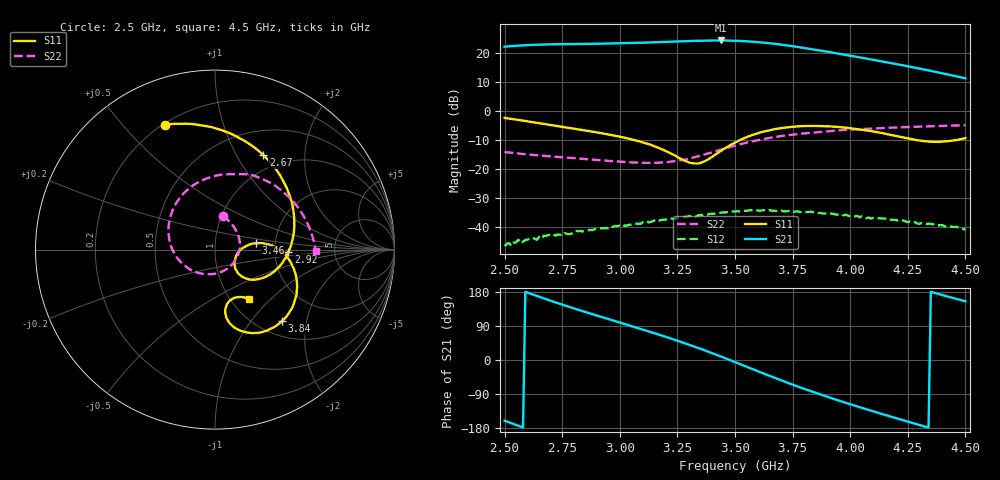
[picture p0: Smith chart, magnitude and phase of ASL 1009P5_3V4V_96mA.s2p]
!ASL 1009P5 : Low Noise Amplifier S-parameter data 2.5-4.5 GHz
!Bias conditions Vd1=3V, Vd2=4V, Total current=96 mA
!Date: Tuesday, January 09, 2007 14:22:50
!S2P File: Measurements: S11, S21, S12, S22:
# Hz S  dB  R 50
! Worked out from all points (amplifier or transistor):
!   201 points, 2.5 GHz to 4.5 GHz, reference 50 ohm
!   highest |S21| = 24.2 dB at 3.44 GHz (marker M1)
!   |S21| within 3 dB of that: start of sweep to 3.833 GHz
!   unconditionally stable (mu >= 1): start of sweep to end of sweep
!   at 2.83 GHz: K = 3.30, MAG = 24.1 dB, |S12| = -41.4 dB
!   at 3.5 GHz: K = 1.64, MAG = 24.8 dB, |S12| = -34.8 dB
!   at 4.5 GHz: K = 9.42, MAG = 13.4 dB, |S12| = -41.1 dB
!   S11 on the Smith chart (normalised r, x): 2.5 GHz: 0.21, +0.66; 2.67 GHz: 0.80, +1.30; 2.92 GHz: 2.38, -0.08; 3.46 GHz: 1.58, +0.12; 3.84 GHz: 1.27, -1.44; 4.5 GHz: 1.21, -0.76
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2.5e9  -2.51 111.8  22.06 -160.3  -46.71 121.9  -14.25 76.8
2.59e9  -3.56 86.0  22.57 179.8  -44.59 102.7  -15.02 64.5
2.67e9  -4.56 62.9  22.81 162.7  -43.10 85.0  -15.55 53.0
2.74e9  -5.46 43.3  22.93 148.3  -42.76 70.6  -16.01 42.3
2.84e9  -6.70 17.0  23.01 128.7  -41.67 56.2  -16.60 24.0
2.92e9  -7.76 -1.9  23.09 113.7  -40.51 42.8  -17.14 7.8
3.04e9  -9.65 -26.1  23.31 91.5  -39.32 22.0  -17.77 -22.7
3.17e9  -12.88 -43.9  23.64 66.9  -37.97 -1.4  -17.97 -64.6
3.25e9  -15.97 -43.7  23.88 50.9  -36.86 -15.6  -17.28 -95.1
3.31e9  -18.04 -28.5  24.04 38.3  -36.29 -29.0  -16.34 -118.3
3.38e9  -16.93 -0.6  24.17 22.9  -35.83 -41.8  -14.82 -144.9
3.44e9  -13.81 8.8  24.21 9.0  -35.13 -57.1  -13.39 -166.6
3.46e9  -12.79 8.9  24.18 4.2  -35.08 -60.9  -12.92 -173.5
3.5e9  -10.97 6.6  24.12 -5.5  -34.78 -69.8  -12.03 173.1
3.58e9  -8.26 -3.7  23.76 -25.0  -34.60 -90.2  -10.49 148.2
3.67e9  -6.40 -18.8  23.08 -46.7  -34.50 -111.7  -9.09 123.3
3.74e9  -5.64 -30.7  22.35 -62.8  -34.47 -126.9  -8.34 106.0
3.84e9  -5.28 -47.0  21.12 -84.6  -35.04 -149.3  -7.54 84.8
4e9  -6.01 -67.9  18.96 -116.7  -36.33 -179.5  -6.52 57.3
4.17e9  -8.25 -80.4  16.51 -148.3  -37.53 151.3  -5.89 34.0
4.34e9  -10.65 -72.5  13.89 -178.4  -38.93 125.0  -5.39 14.7
4.5e9  -9.48 -55.5  11.15 155.0  -41.06 98.0  -5.03 -1.0
